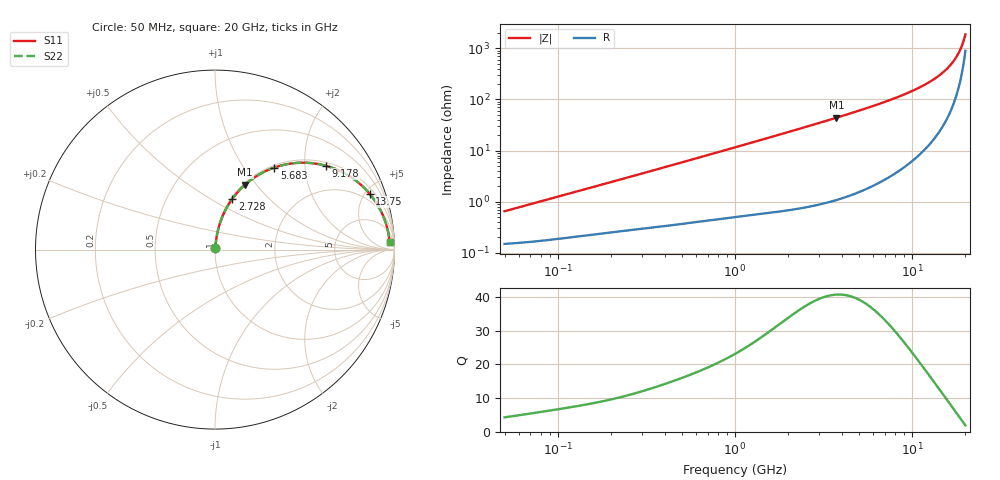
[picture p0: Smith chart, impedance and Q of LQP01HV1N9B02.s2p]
!Murata Part Number: LQP01HV1N9B02
!These Parameters are Measured in Series Mode Connection
!  o--[Z]--o
!Port1  Port2
!  o-------o
!Freq. Start=50[MHz] Stop=20[GHz], 401[Steps]
# Hz S RI R 50
!Freq.(Hz) S11(Real) S11(Imag) S21(Real) S21(Imag) S12(Real) S12(Imag) S22(Real) S22(Imag)
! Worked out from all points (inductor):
!   401 points, 50 MHz to 20 GHz, reference 50 ohm
!   read as one part in series: L = 2.01 nH near 51.52 MHz
!   highest Q = 40.7 at 3.736 GHz (marker M1), where L = 1.87 nH
!   S11 on the Smith chart (normalised r, x): 50 MHz: 1.00, +0.01; 2.728 GHz: 1.02, +0.63; 5.683 GHz: 1.04, +1.39; 9.178 GHz: 1.10, +2.56; 13.75 GHz: 1.39, +5.38; 20 GHz: 19, +33
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5e7  0.00153 0.00633  0.9985 -0.00633  0.9985 -0.00633  0.00153 0.00633
1.364002e8  0.00242 0.0167  0.9976 -0.0167  0.9976 -0.0167  0.00242 0.0167
3.721004e8  0.00513 0.0435  0.9949 -0.0435  0.9949 -0.0435  0.00513 0.0435
6.285508e8  0.00932 0.0722  0.9907 -0.0722  0.9907 -0.0722  0.00932 0.0722
1e9  0.0179 0.1128  0.9821 -0.1128  0.9821 -0.1128  0.0179 0.1128
1.766834e9  0.0452 0.1927  0.9548 -0.1927  0.9548 -0.1927  0.0452 0.1927
2.728004e9  0.0967 0.2828  0.9033 -0.2828  0.9033 -0.2828  0.0967 0.2828
3.736399e9  0.1672 0.3611  0.8328 -0.3611  0.8328 -0.3611  0.1672 0.3611
4.608136e9  0.2375 0.4132  0.7625 -0.4132  0.7625 -0.4132  0.2375 0.4132
5.683258e9  0.3303 0.4571  0.6697 -0.4571  0.6697 -0.4571  0.3303 0.4571
7.442007e9  0.4822 0.4842  0.5178 -0.4842  0.5178 -0.4842  0.4822 0.4842
9.178299e9  0.6176 0.4671  0.3824 -0.4671  0.3824 -0.4671  0.6176 0.4671
1.149051e10  0.762 0.4007  0.238 -0.4007  0.238 -0.4007  0.762 0.4007
1.257102e10  0.8146 0.3595  0.1854 -0.3595  0.1854 -0.3595  0.8146 0.3595
1.375312e10  0.8618 0.3105  0.1382 -0.3105  0.1382 -0.3105  0.8618 0.3105
1.550395e10  0.9141 0.2344  0.0859 -0.2344  0.0859 -0.2344  0.9141 0.2344
1.646126e10  0.9347 0.1926  0.0653 -0.1926  0.0653 -0.1926  0.9347 0.1926
1.721783e10  0.9476 0.1598  0.0524 -0.1598  0.0524 -0.1598  0.9476 0.1598
1.800918e10  0.9581 0.126  0.0419 -0.126  0.0419 -0.126  0.9581 0.126
1.855685e10  0.9637 0.1031  0.0363 -0.1031  0.0363 -0.1031  0.9637 0.1031
1.970266e10  0.9716 0.0565  0.0284 -0.0565  0.0284 -0.0565  0.9716 0.0565
2e10  0.9728 0.0447  0.0272 -0.0447  0.0272 -0.0447  0.9728 0.0447
